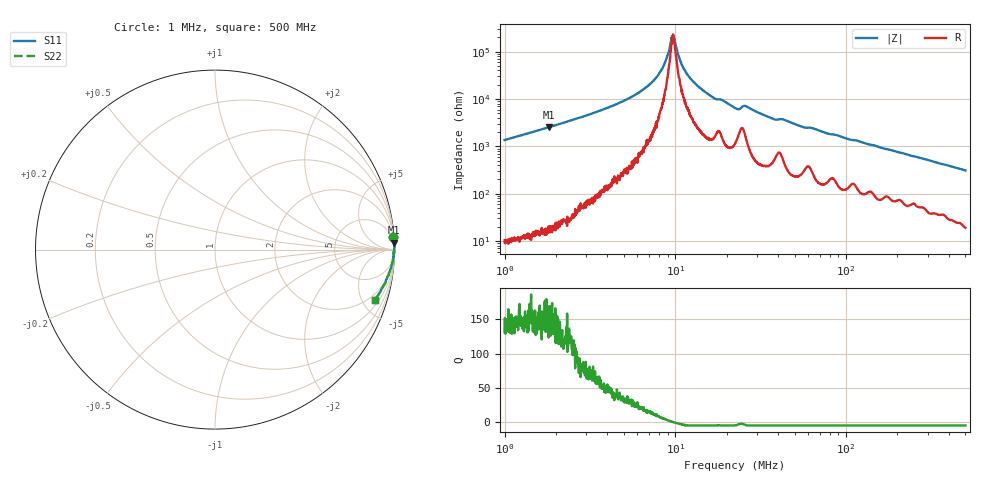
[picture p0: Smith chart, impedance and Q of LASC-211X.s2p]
!s-Parameter Generated by FASTRON Sdn. Bhd.
!FASTRON P/N : LASC-211X
!Keysight Technologies,E4991B,MY54100416,A.01.15
!Date: Thu Mar 19 08:56:17 2026
!Version  : Rev00 Thu Mar 19 08:56:17 2026
!Data & Calibration Information:
!PortZ  Port1:50+j0  Port2:50+j0
!When reading, reference impedance value at option line is always used.
!Remarks : This data is being provided solely for informational purposes.
!Freq	S11	S21	S12	S22
# Hz S dB R 50
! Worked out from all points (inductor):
!   1601 points, 1 MHz to 500 MHz, reference 50 ohm
!   read as one part in series: L = 214 uH near 1.032 MHz
!   highest Q = 158 at 1.826 MHz (marker M1), where L = 222 uH
!   self-resonance near 9.663 MHz
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1000000  -0.03 4.2  -22.72 -85.4  -22.72 -85.4  -0.03 4.2
1825840  -0.01 2.2  -28.15 -87.4  -28.15 -87.4  -0.01 2.2
2820919  -0.01 1.4  -32.38 -87.9  -32.38 -87.9  -0.01 1.4
5566606  -0.00 0.5  -40.94 -87.0  -40.94 -87.0  -0.00 0.5
6946104  -0.00 0.3  -45.69 -86.0  -45.69 -86.0  -0.00 0.3
7957584  -0.00 0.2  -50.23 -83.4  -50.23 -83.4  -0.00 0.2
8701196  -0.00 0.1  -55.35 -75.3  -55.35 -75.3  -0.00 0.1
9477412  -0.00 0.0  -65.74 -40.3  -65.74 -40.3  -0.00 0.0
9700875  -0.00 -0.0  -67.25 6.0  -67.25 6.0  -0.00 -0.0
9891114  -0.00 -0.0  -65.30 31.3  -65.30 31.3  -0.00 -0.0
1.052531e7  -0.00 -0.1  -57.53 68.2  -57.53 68.2  -0.00 -0.1
1.098475e7  -0.00 -0.1  -54.02 75.0  -54.02 75.0  -0.00 -0.1
1.248696e7  -0.01 -0.2  -47.97 80.7  -47.97 80.7  -0.01 -0.2
1.6645e7  -0.01 -0.5  -40.59 81.9  -40.59 81.9  -0.01 -0.5
2.236068e7  -0.02 -0.9  -36.24 78.9  -36.24 78.9  -0.02 -0.9
2.581658e7  -0.03 -0.8  -37.06 76.4  -37.06 76.4  -0.03 -0.8
3.748322e7  -0.03 -1.5  -31.60 81.2  -31.60 81.2  -0.03 -1.5
4.260918e7  -0.04 -1.5  -31.47 80.2  -31.47 80.2  -0.04 -1.5
5.570526e7  -0.04 -2.2  -28.22 81.6  -28.22 81.6  -0.04 -2.2
6.307767e7  -0.05 -2.3  -27.81 80.8  -27.81 80.8  -0.05 -2.3
1.77937e8  -0.15 -6.5  -18.83 77.9  -18.83 77.9  -0.15 -6.5
5e8  -0.58 -17.5  -10.43 69.0  -10.43 69.0  -0.58 -17.5
